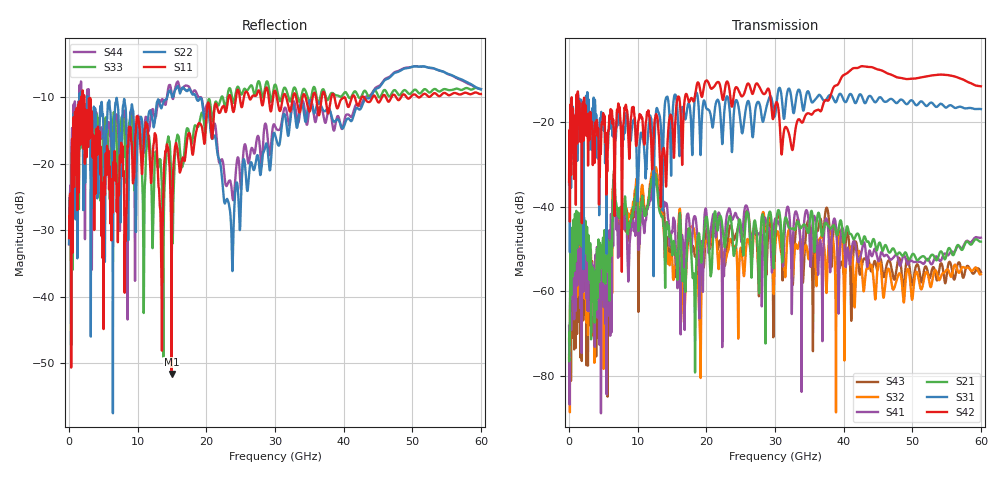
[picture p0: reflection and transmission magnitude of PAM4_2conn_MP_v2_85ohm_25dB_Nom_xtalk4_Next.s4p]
! Info: Touchstone file created by Circ.  Input file=FAB50GbE_2conn_Midplane_Examax_Topo2_v2_85ohm_25dB_Nom.circ
# Hz S RI R 50
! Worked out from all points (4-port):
!   6000 points, 10 MHz to 60 GHz, reference 50 ohm
!   strongest paths, dB at 10 MHz, 15.01 GHz, 30.01 GHz, 45.01 GHz, 60 GHz:
!     S42: -34.0, -19.7, -16.3, -7.5, -11.4
!     S31: -34.6, -21.2, -18.4, -14.5, -16.8
!     S21: -75.9, -50.5, -47.5, -49.4, -48.2
!     S41: -68.1, -45.9, -42.9, -52.6, -47.3
!     S32: -75.1, -51.7, -50.4, -53.5, -55.9
!     S43: -71.2, -48.8, -47.6, -54.5, -55.4
!   lowest |S11| = -51.6 dB at 14.93 GHz (marker M1), VSWR 1.01, Z = 50.3 - j0.0672 ohm
!   |S11| at or under -10 dB: start of sweep to 1.766 GHz; 2.214 GHz to 23.25 GHz (21.03 GHz wide, 165 % of centre); 38.66 GHz to 41.24 GHz (2.581 GHz wide, 6.46 % of centre)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
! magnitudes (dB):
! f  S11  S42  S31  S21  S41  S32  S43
! 10 MHz  -31.2  -34.0  -34.6  -75.9  -68.1  -75.1  -71.2
! 870 MHz  -12.3  -20.6  -22.2  -41.6  -48.3  -48.5  -54.2
! 5.55 GHz  -17.5  -31.3  -25.9  -48.9  -54.2  -55.8  -56.2
! 6.63 GHz  -18.2  -42.1  -23.4  -31.4  -34.7  -31.4  -32.9
! 14.93 GHz  -51.6  -18.5  -27.1  -48.5  -45.9  -51.2  -48.8
! 23.76 GHz  -11.5  -16.2  -26.7  -45.9  -43.0  -48.5  -45.4
! 60 GHz  -9.6  -11.4  -16.8  -48.2  -47.3  -55.9  -55.4
